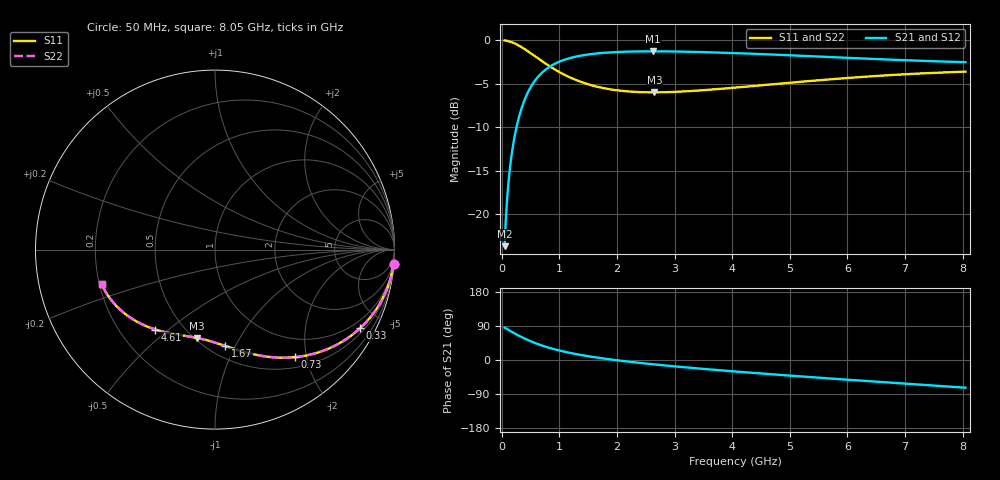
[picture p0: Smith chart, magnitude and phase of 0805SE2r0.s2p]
! AVX Thin Film Operation		Date: August 2001
! Description: Accu-P® Series, Thin Film, SMD, RF Capacitor
! Part Number: 08051J2R0ABT
! 50 MHz  -  8.05 GHz
! Serial Measurements
# mhz S db R 50
!	S11		S21		S12		S22
!	dB	Phase	dB	Phase	dB	Phase	dB	Phase
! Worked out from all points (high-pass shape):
!   401 points, 50 MHz to 8.05 GHz, reference 50 ohm
!   highest |S21| = -1.27 dB at 2.63 GHz (marker M1); lowest = -23.7 dB at 50 MHz (marker M2)
!   |S21| within 3 dB of the highest: 621.2 MHz to end of sweep
!   lowest |S11| = -6.0 dB at 2.65 GHz (marker M3), VSWR 3.02, Z = 25.7 - j33.8 ohm
!   |S11| at or under -10 dB: nowhere
!   |S22| runs from -6.0 to 0.0 dB; largest |S21 - S12| = 0
!   S11 on the Smith chart (normalised r, x): 50 MHz: 1, -25; 330 MHz: 0.68, -3.84; 730 MHz: 0.66, -1.80; 1.67 GHz: 0.60, -0.91; 4.61 GHz: 0.35, -0.45; 8.05 GHz: 0.21, -0.14
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50  -0.02 -4.6  -23.66 85.4  -23.66 85.4  -0.02 -4.6
70  -0.04 -6.4  -20.76 83.6  -20.76 83.6  -0.04 -6.4
130  -0.12 -11.8  -15.48 78.2  -15.48 78.2  -0.12 -11.8
170  -0.21 -15.3  -13.25 74.7  -13.25 74.7  -0.21 -15.3
250  -0.44 -22.1  -10.17 67.9  -10.17 67.9  -0.44 -22.1
330  -0.73 -28.4  -8.11 61.6  -8.11 61.6  -0.73 -28.4
410  -1.06 -34.3  -6.63 55.6  -6.63 55.6  -1.06 -34.4
510  -1.52 -41.0  -5.31 48.9  -5.31 48.9  -1.52 -41.1
730  -2.54 -53.4  -3.54 36.6  -3.54 36.6  -2.54 -53.4
1030  -3.76 -66.0  -2.38 24.0  -2.38 24.0  -3.76 -66.0
1390  -4.82 -77.1  -1.74 12.9  -1.74 12.9  -4.82 -77.1
1670  -5.36 -83.9  -1.50 6.1  -1.50 6.1  -5.36 -83.9
2090  -5.81 -92.3  -1.32 -2.4  -1.32 -2.4  -5.81 -92.4
2630  -5.98 -101.3  -1.27 -11.4  -1.27 -11.4  -5.98 -101.3
2650  -5.98 -101.6  -1.27 -11.7  -1.27 -11.7  -5.98 -101.6
2730  -5.98 -102.8  -1.27 -12.9  -1.27 -12.9  -5.98 -102.8
3370  -5.79 -111.7  -1.33 -21.8  -1.33 -21.8  -5.79 -111.7
4050  -5.44 -120.2  -1.47 -30.3  -1.47 -30.3  -5.44 -120.3
4610  -5.11 -126.7  -1.61 -36.8  -1.61 -36.8  -5.11 -126.8
5390  -4.65 -135.3  -1.83 -45.5  -1.83 -45.5  -4.65 -135.4
6730  -4.01 -149.4  -2.22 -59.5  -2.22 -59.5  -4.01 -149.4
8050  -3.60 -162.9  -2.51 -73.1  -2.51 -73.1  -3.60 -163.0
